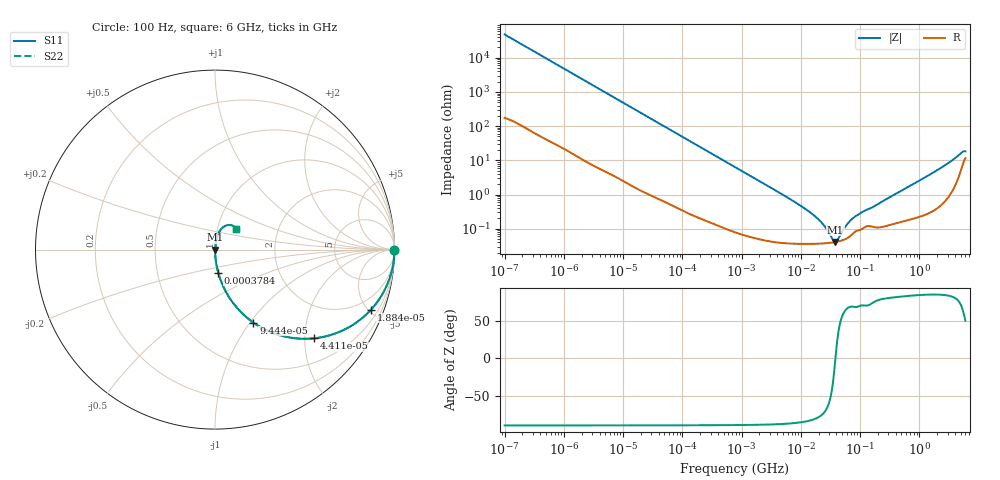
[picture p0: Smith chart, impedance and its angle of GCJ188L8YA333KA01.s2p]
!Murata Part Number: GCJ188L8YA333KA01
!These Parameters are Measured in Series Mode Connection
!Data Generated on Mar 13, 2026
!  o--ll--o
!Port1  Port2
!  o------o
!Operation Temp=25[degC], DC Bias Voltage=0[V]
!Freq. Start=100[Hz] Stop=6[GHz] 401[Steps]
# Hz S RI R 50
!Freq.(Hz) S11(Real) S11(Imag) S21(Real) S21(Imag) S12(Real) S12(Imag) S22(Real) S22(Imag)
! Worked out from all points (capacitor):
!   401 points, 100 Hz to 6 GHz, reference 50 ohm
!   read as one part in series: C = 33.1 nF near 109 Hz
!   lowest |Z| = 40.9 mohm at 38.09 MHz (marker M1)
!   series resonance near 38.39 MHz, so ESL is about 520 pH
!   S11 on the Smith chart (normalised r, x): 100 Hz: open; 18.84 kHz: 1.03, -5.18; 44.11 kHz: 1.01, -2.22; 94.44 kHz: 1.01, -1.04; 378.4 kHz: 1.00, -0.26; 6 GHz: 1.23, +0.28
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100  1 -0.00208  1.19e-05 0.00208  1.19e-05 0.00208  1 -0.00208
2008  0.9981 -0.0413  0.0019 0.0413  0.0019 0.0413  0.9981 -0.0413
6728  0.9806 -0.1355  0.0194 0.1355  0.0194 0.1355  0.9806 -0.1355
18841  0.869 -0.3348  0.131 0.3348  0.131 0.3348  0.869 -0.3348
40335  0.5949 -0.4879  0.4051 0.4879  0.4051 0.4879  0.5949 -0.4879
44113  0.5515 -0.4943  0.4485 0.4943  0.4485 0.4943  0.5515 -0.4943
94437  0.2144 -0.407  0.7856 0.407  0.7856 0.407  0.2144 -0.407
169018  0.0799 -0.2673  0.9201 0.2673  0.9201 0.2673  0.0799 -0.2673
378399  0.018 -0.128  0.982 0.128  0.982 0.128  0.018 -0.128
774597  0.00485 -0.0636  0.9951 0.0636  0.9951 0.0636  0.00485 -0.0636
6353432  0.000429 -0.00764  0.9996 0.00764  0.9996 0.00764  0.000429 -0.00764
1.555665e7  0.000369 -0.00269  0.9996 0.00269  0.9996 0.00269  0.000369 -0.00269
2.327686e7  0.000373 -0.00136  0.9996 0.00136  0.9996 0.00136  0.000373 -0.00136
3.482834e7  0.000398 -0.000254  0.9996 0.000254  0.9996 0.000254  0.000398 -0.000254
3.80911e7  0.000408 -1.99e-05  0.9996 1.99e-05  0.9996 1.99e-05  0.000408 -1.99e-05
4.165952e7  0.000421 0.000215  0.9996 -0.000215  0.9996 -0.000215  0.000421 0.000215
5.960426e7  0.000522 0.0012  0.9995 -0.0012  0.9995 -0.0012  0.000522 0.0012
7.797396e7  0.000758 0.00199  0.9992 -0.00199  0.9992 -0.00199  0.000758 0.00199
3.124326e8  0.00134 0.00816  0.9987 -0.00816  0.9987 -0.00816  0.00134 0.00816
3.205649e9  0.0163 0.0844  0.9837 -0.0844  0.9837 -0.0844  0.0163 0.0844
5.016141e9  0.0669 0.1358  0.9331 -0.1358  0.9331 -0.1358  0.0669 0.1358
6e9  0.1187 0.112  0.8813 -0.112  0.8813 -0.112  0.1187 0.112
